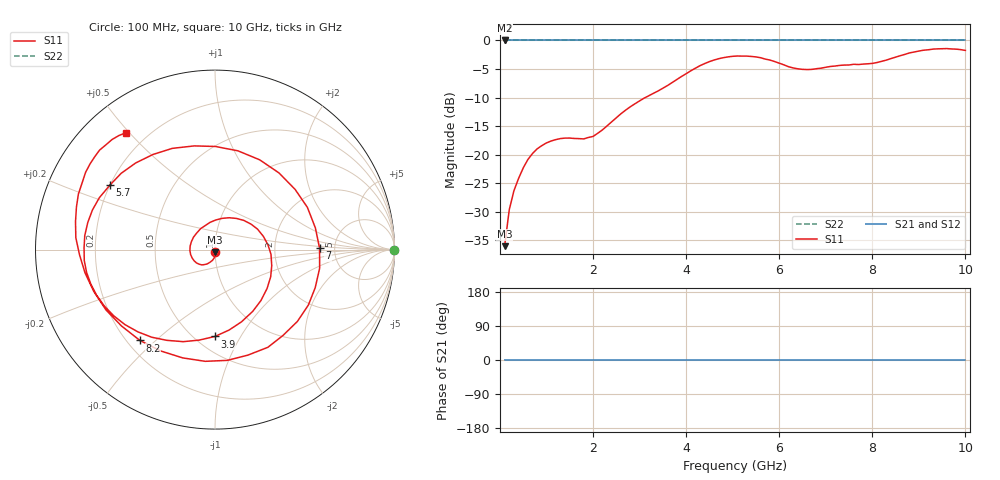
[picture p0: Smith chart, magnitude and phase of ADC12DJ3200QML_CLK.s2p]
!	Texas	"Instruments,"	Inc.
!	ADC12DJ3200	-	CLK		S-Parameters	(DES	"Mode,"	Fs	=	3.2	"GSPS,"	25	degC	"case,"	15	degC	juntion)
!	Port	1	represents	the	100-ohm	differential	"input,"	Port	2	the	digital	output
!	freq	dbS11	angS11	dbS21	angS21	dbS12	angS12	dbS22	angS22
#	HZ	S	DB	R	100
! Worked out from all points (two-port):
!   100 points, 100 MHz to 10 GHz, reference 100 ohm
!   highest |S21| = 0.00 dB at 100 MHz (marker M1); lowest = 0.0 dB at 100 MHz (marker M2)
!   |S21| within 3 dB of the highest: start of sweep to end of sweep
!   lowest |S11| = -36.0 dB at 100 MHz (marker M3), VSWR 1.03, Z = 100 - j3.16 ohm
!   |S11| at or under -10 dB: start of sweep to 3.12 GHz
!   |S22| runs from 0.0 to 0.0 dB; largest |S21 - S12| = 0
!   S11 on the Smith chart (normalised r, x): 100 MHz: 1.00, -0.03; 3.9 GHz: 0.62, -0.78; 5.7 GHz: 0.20, +0.27; 7 GHz: 3.79, +0.09; 8.2 GHz: 0.25, -0.45; 10 GHz: 0.12, +0.49
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1e8  -36.00 -83.8  0.00 0.0  0.00 0.0  0.00 0.0
2e8  -29.62 -89.3  0.00 0.0  0.00 0.0  0.00 0.0
3e8  -26.30 -96.6  0.00 0.0  0.00 0.0  0.00 0.0
6e8  -20.83 -118.6  0.00 0.0  0.00 0.0  0.00 0.0
1.1e9  -17.59 -151.7  0.00 0.0  0.00 0.0  0.00 0.0
1.8e9  -17.23 137.4  0.00 0.0  0.00 0.0  0.00 0.0
2.6e9  -12.82 45.4  0.00 0.0  0.00 0.0  0.00 0.0
3.4e9  -8.83 -36.7  0.00 0.0  0.00 0.0  0.00 0.0
3.9e9  -6.31 -90.0  0.00 0.0  0.00 0.0  0.00 0.0
4.4e9  -4.04 -133.1  0.00 0.0  0.00 0.0  0.00 0.0
5.1e9  -2.72 -175.2  0.00 0.0  0.00 0.0  0.00 0.0
5.7e9  -3.26 148.5  0.00 0.0  0.00 0.0  0.00 0.0
6.2e9  -4.59 101.3  0.00 0.0  0.00 0.0  0.00 0.0
6.7e9  -5.06 37.0  0.00 0.0  0.00 0.0  0.00 0.0
7e9  -4.69 0.8  0.00 0.0  0.00 0.0  0.00 0.0
7.3e9  -4.36 -30.7  0.00 0.0  0.00 0.0  0.00 0.0
7.7e9  -4.21 -72.8  0.00 0.0  0.00 0.0  0.00 0.0
8.2e9  -3.65 -129.6  0.00 0.0  0.00 0.0  0.00 0.0
8.4e9  -3.17 -151.1  0.00 0.0  0.00 0.0  0.00 0.0
8.8e9  -2.18 175.1  0.00 0.0  0.00 0.0  0.00 0.0
9.2e9  -1.63 153.2  0.00 0.0  0.00 0.0  0.00 0.0
1e10  -1.74 127.1  0.00 0.0  0.00 0.0  0.00 0.0
